(* Logix 5000 Rung export; software revision 16.03 *)

TYPE GSCDATETIME :   // Stores the date and time value
STRUCT
   Year : DINT;
   Month : DINT;
   Day : DINT;
   Hour : DINT;
   Minute : DINT;
   Seconds : DINT;
END_STRUCT
END_TYPE

TYPE GSCETHERNET :   // Stores the MVI56E-GSC IP settings
STRUCT
   IP : INT[4];
   Netmask : INT[4];
   Gateway : INT[4];
END_STRUCT
END_TYPE

TYPE GSCETHERNETTYPE :   // Allows read/write Ethernet settings between the module and processor
STRUCT
   Read : BOOL;   // Enable Ethernet configuration transfer from module to processor
   Write : BOOL;   // Enable Ethernet configuration transfer from processor to module
   Config : GSCETHERNET;
END_STRUCT
END_TYPE

TYPE GSCCLOCKTYPE :   // Allows read/write of clock value between the module and processor
STRUCT
   Read : BOOL;   // Reads current time from the module
   Write : BOOL;   // Writes current time from the module
   Config : GSCDATETIME;   // Date and time configuration read or written between the module and processor
END_STRUCT
END_TYPE

ADD_ON_INSTRUCTION AOI56EGSC_OPTIONAL   (* revision 1.1 *)
// MVI56E-GSC Optional Add-On Ethernet/Clock
// Revision note:
// Added viewing capability for the Add_On Instruction
VAR_IN_OUT
   MVI56EGSCEthernet : GSCETHERNETTYPE; {required}   // MVI56E-GSC Rev2 Ethernet Settings
   MVI56EGSCClock : GSCCLOCKTYPE; {required}   // MVI56E-GSC Rev2 Clock Settings
   ReadEthernetMSG : MESSAGE; {required}   // Read Ethernet Settings Message
   WriteEthernetMSG : MESSAGE; {required}   // Write Ethernet Settings Message
   ReadClockMSG : MESSAGE; {required}   // Read Clock Settings Message
   WriteClockMSG : MESSAGE; {required}   // Write Clock Settings Message
END_VAR

ROUTINE Logic   (* ladder *)
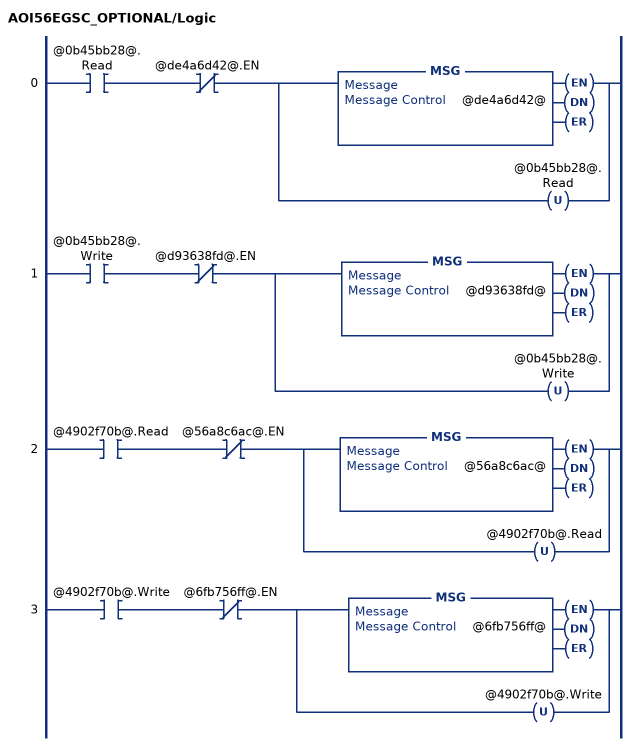
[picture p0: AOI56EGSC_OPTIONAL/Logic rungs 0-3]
   0: XIC(@0b45bb28@.Read)XIO(@de4a6d42@.EN)[MSG(@de4a6d42@) ,OTU(@0b45bb28@.Read) ];
   1: XIC(@0b45bb28@.Write)XIO(@d93638fd@.EN)[MSG(@d93638fd@) ,OTU(@0b45bb28@.Write) ];
   2: XIC(@4902f70b@.Read)XIO(@56a8c6ac@.EN)[MSG(@56a8c6ac@) ,OTU(@4902f70b@.Read) ];
   3: XIC(@4902f70b@.Write)XIO(@6fb756ff@.EN)[MSG(@6fb756ff@) ,OTU(@4902f70b@.Write) ];
END_ROUTINE
END_ADD_ON_INSTRUCTION

VAR_GLOBAL   (* controller tags *)
   AOI56EGSC_OPTIONAL : AOI56EGSC_OPTIONAL;
   MVI56EGSCEthernet : GSCETHERNETTYPE;
   ReadClockMSG : MESSAGE;
        MessageParameters(MessageType := CIP Generic, ConnectedFlag := 2, ConnectionPath := GSC, ServiceCode := 16#000e, ObjectType := 16#0004, TargetObject := 8, AttributeNumber := 16#0020, DestinationTag := MVI56EGSCClock.Config)
   WriteEthernetMSG : MESSAGE;
        MessageParameters(MessageType := CIP Generic, RequestedLength := 24, ConnectedFlag := 2, ConnectionPath := GSC, ServiceCode := 16#0010, ObjectType := 16#0004, TargetObject := 8, LocalElement := MVI56EGSCEthernet.Config)
   WriteClockMSG : MESSAGE;
        MessageParameters(MessageType := CIP Generic, RequestedLength := 24, ConnectedFlag := 2, ConnectionPath := GSC, ServiceCode := 16#0010, ObjectType := 16#0004, TargetObject := 8, AttributeNumber := 16#0020, LocalElement := MVI56EGSCClock.Config)
   ReadEthernetMSG : MESSAGE;
        MessageParameters(MessageType := CIP Generic, ConnectedFlag := 2, ConnectionPath := GSC, ServiceCode := 16#000e, ObjectType := 16#0004, TargetObject := 8, DestinationTag := MVI56EGSCEthernet.Config)
   MVI56EGSCClock : GSCCLOCKTYPE;
END_VAR

PROGRAM MainProgram

ROUTINE MainRoutine   (* ladder *)
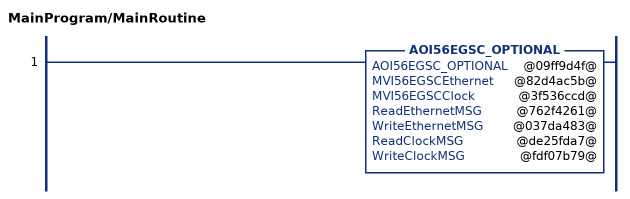
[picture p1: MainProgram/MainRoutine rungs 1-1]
   1: AOI56EGSC_OPTIONAL(@09ff9d4f@,@82d4ac5b@,@3f536ccd@,@762f4261@,@037da483@,@de25fda7@,@fdf07b79@);
END_ROUTINE
END_PROGRAM
